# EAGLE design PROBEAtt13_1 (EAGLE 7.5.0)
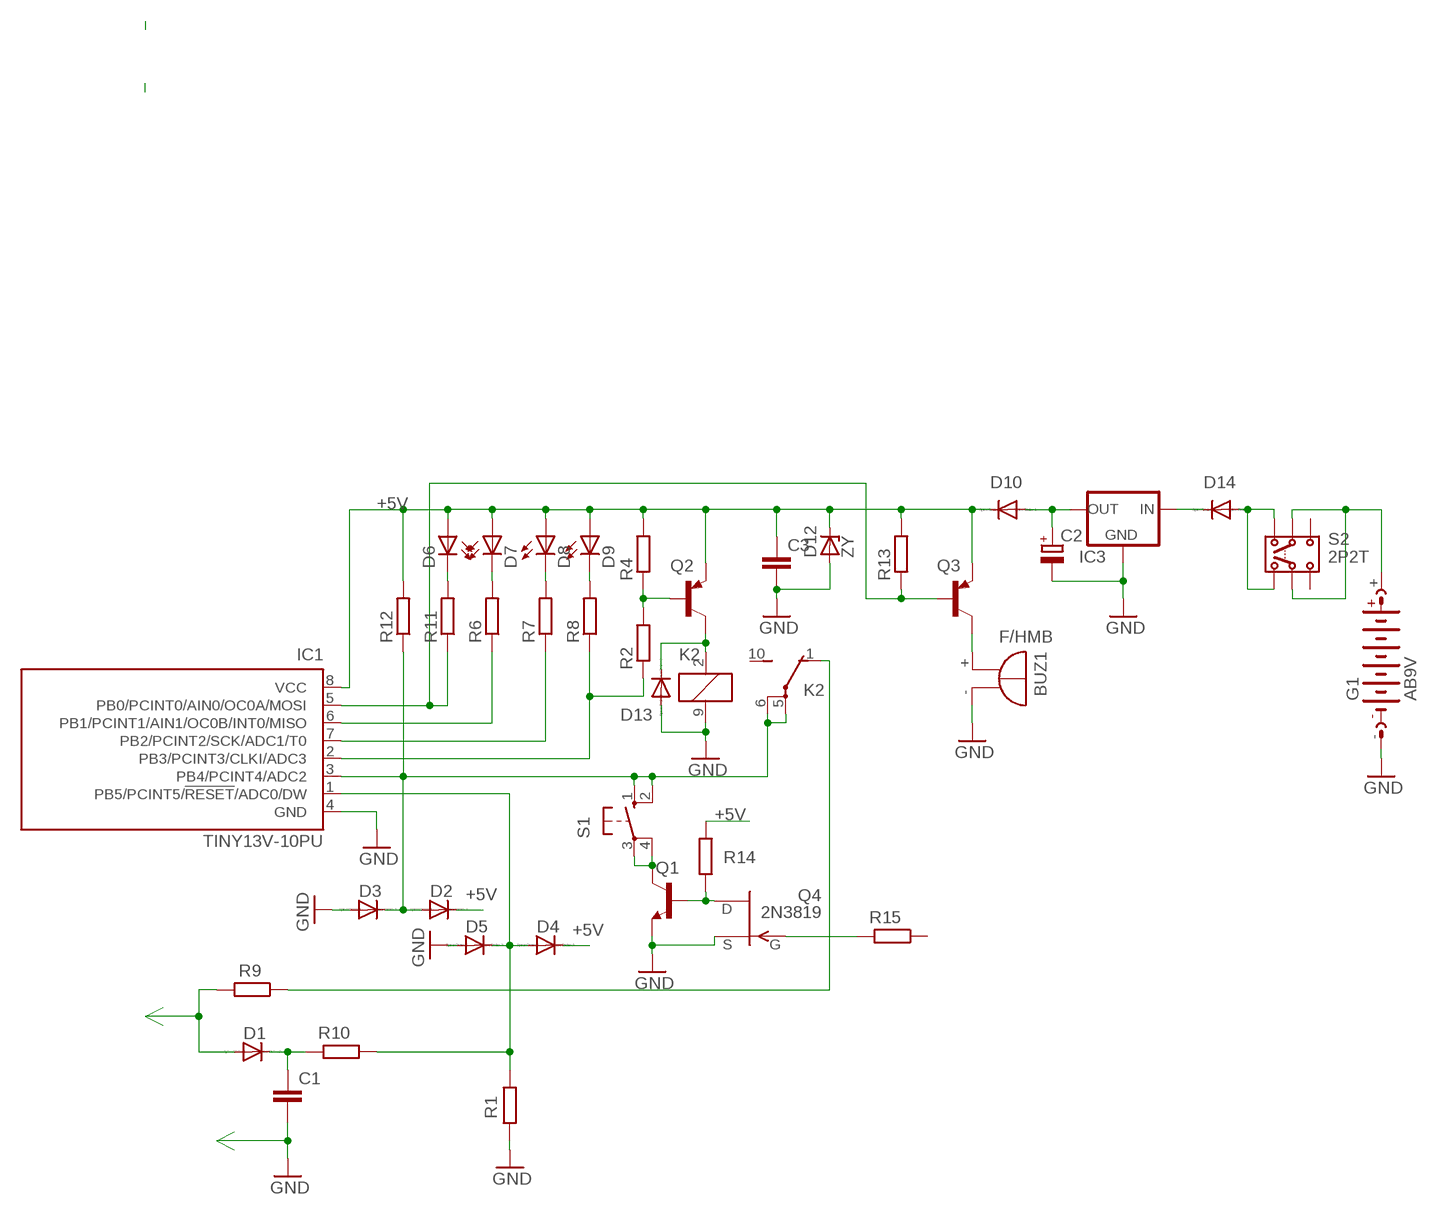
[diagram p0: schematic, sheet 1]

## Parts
BUZ1  F/HMB  [F/HMB]
C1  C-EU150-091X182  [C150-091X182]
C2  CPOL-EUE5-10.5  [E5-10,5]
C3  C-EUC1206  [C1206]
D1  1N4004  [DO41-10]
D2  1N4004  [DO41-10]
D3  1N4004  [DO41-10]
D4  1N4004  [DO41-10]
D5  1N4004  [DO41-10]
D6  LED5MM  [LED5MM]
D7  LED5MM  [LED5MM]
D8  LED5MM  [LED5MM]
D9  LED5MM  [LED5MM]
D10  1N4004  [DO41-10]
D12  ZY  [P1Z12]
D13  1N4004  [DO41-10]
D14  1N4004  [DO41-10]
G1  AB9V  [AB9V]
IC1  TINY13V-10PU  [DIL08]
IC3  78XXL  [78XXL]
K2  G5V1  [G5V1]
Q1  BC337  [TO92]
Q2  BC327  [TO92]
Q3  BC327  [TO92]
Q4  2N3819  [TO92]
R1  R-EU_0207/10  [0207/10]
R2  R-EU_0207/10  [0207/10]
R4  R-EU_0204/7  [0204/7]
R6  R-EU_0204/7  [0204/7]
R7  R-EU_0204/7  [0204/7]
R8  R-EU_0207/12  [0207/12]
R9  R-EU_0617/22  [0617/22]
R10  R-EU_0617/22  [0617/22]
R11  R-EU_0204/7  [0204/7]
R12  R-EU_0204/7  [0204/7]
R13  R-EU_0204/7  [0204/7]
R14  R-EU_0204/7  [0204/7]
R15  R-EU_0204/7  [0204/7]
S1  10-XX  [B3F-10XX]
S2  2P2T  [2P2T]

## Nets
+5V: C3.1 D2.C D4.C D6.A D7.A D8.A D9.A D10.C D12.C IC1.8(VCC) Q2.1(E) Q3.1(E) R4.2 R12.2 R13.2 R14.1
GND: BUZ1.- C1.2 C2.- C3.2 D3.A D5.A D12.A D13.A G1.- IC1.4(GND) IC3.GND K2.9 Q1.1(E) Q4.3(S) R1.2
N$1: IC1.5(PB0/PCINT0/AIN0/OC0A/MOSI) Q3.2(B) R11.1 R13.1
N$2: D6.K(C) R11.2
N$3: D2.A D3.C IC1.3(PB4/PCINT4/ADC2) K2.5(2:P) K2.6(2:P) R12.1 S1.1(S) S1.2(S1)
N$4: Q1.3(C) S1.3(P) S1.4(P1)
N$5: IC1.6(PB1/PCINT1/AIN1/OC0B/INT0/MISO) R6.1
N$6: D7.K(C) R6.2
N$7: IC1.7(PB2/PCINT2/SCK/ADC1/T0) R7.1
N$8: D8.K(C) R7.2
N$9: D4.A D5.C IC1.1(PB5/PCINT5/!RESET!/ADC0/DW) R1.1 R10.1
N$10: IC1.2(PB3/PCINT3/CLKI/ADC3) R2.1 R8.1
N$11: D9.K(C) R8.2
N$12: D13.C K2.2 Q2.3(C)
N$13: Q1.2(B) Q4.1(D) R14.2
N$14: C2.+ D10.A IC3.OUT
N$15: Q2.2(B) R2.2 R4.1
N$16: K2.1(2:O) R9.1
N$17: D1.A R9.2
N$18: D14.C IC3.IN
N$19: C1.1 D1.C R10.2
N$20: D14.A S2.1.1 S2.1.2
N$21: Q4.2(G) R15.2
N$22: G1.+ S2.2.1 S2.2.2
N$23: BUZ1.+ Q3.3(C)
Unconnected: K2.10(2:S) R15.1 S2.3.1 S2.3.2

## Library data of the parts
BUZ1 = buzzer:F/HMB: BUZZER; OC_FARNELL: unknown; OC_NEWARK: unknown
C1 C3 = rcl:C-EU: CAPACITOR, European symbol
C2 = rcl:CPOL-EU: POLARIZED CAPACITOR, European symbol
D1-D5 D10 D13 D14 = diode:1N4004: DIODE
D6-D9 = led:LED: LED
D12 = diode:ZY: Z DIODE
G1 = battery:AB9V: 9-V BATTERY CLIP
IC1 = atmel:TINY13: 8-bit AVR Microcontroller with 1K Bytes In-System Programmable Flash Source: http://www.atmel.com/dyn/resources/prod_documents/2535S.pdf; MPN: ATTINY13V-10PU; OC_FARNELL: 9171576; OC_NEWARK: 96K6523
IC3 = v-reg:78XXL: VOLTAGE REGULATOR
K2 = relay:G5V1: RELAY 1 x switch, 0.5 A/125 V AC, 1 A/24 V DC , Omron; MPN: G5V-1-DC24; OC_FARNELL: 9949593; OC_NEWARK: 36M6377
Q1 = transistor:BC337: NPN TRANSISTOR
Q2 Q3 = transistor-pnp:BC327: PNP Transistor
Q4 = transistor-fet:2N3819: N-Channel Junction FET
R1 R2 R4 R6-R15 = rcl:R-EU_: RESISTOR, European symbol
S1 = switch-omron:10-XX: OMRON SWITCH; MPN: B3F-1000; OC_FARNELL: 176432; OC_NEWARK: 36M3542
S2 = switch:2P2T: SLIDE SWITCH 2P2T Part No. SS-22F05-G(A)4 Source: CANAL ELECTRONIC CO., LTD .. switsch.pdf

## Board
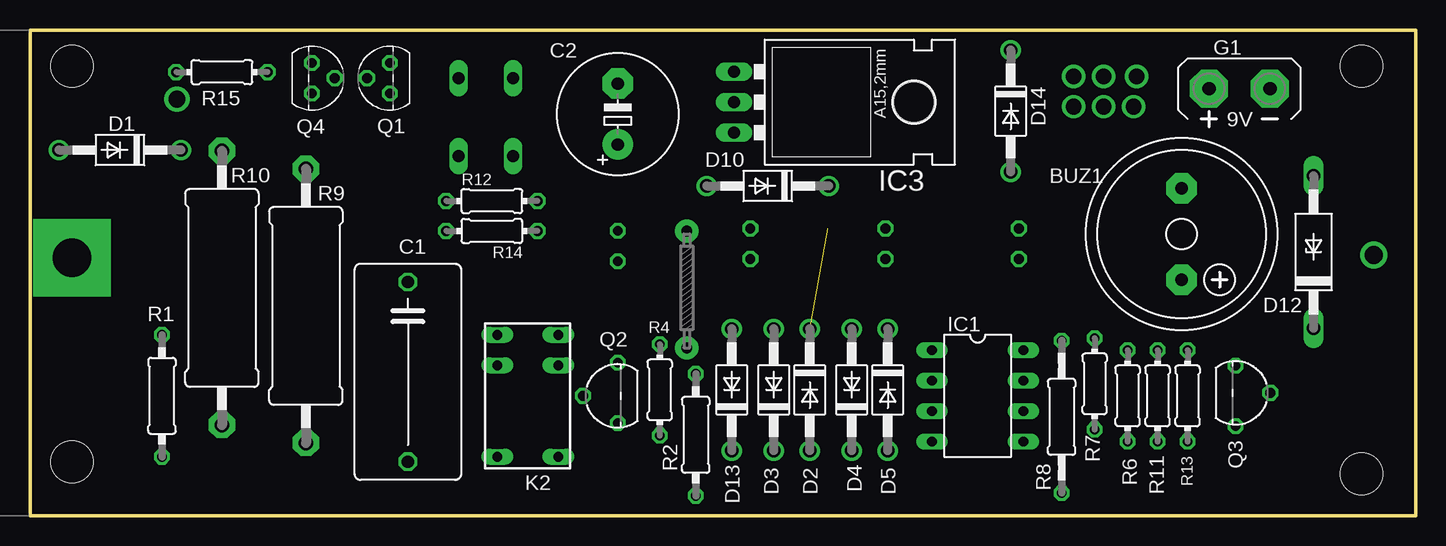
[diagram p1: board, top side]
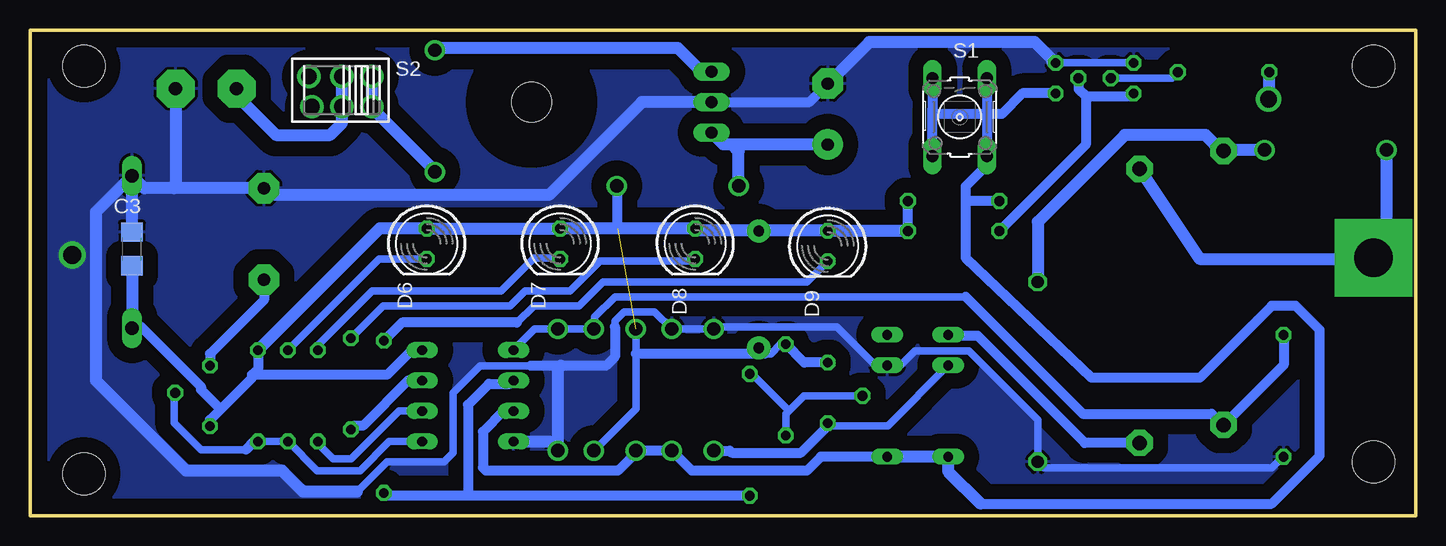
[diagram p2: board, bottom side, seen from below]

Size 115.5 x 40.5 mm. Coordinates in mm from the lower left corner, seen from the top.
Outline: 0,0 0,40.5 115.5,40.5 115.5,0 0,0
Copper layers (1*16): Top 0.035mm / dielectric 1.5mm / Bottom 0.035mm
Design rules "default": minimum track width 10mil, minimum drill 24mil, track to track 8mil, track to pad 8mil, pad to pad 8mil, via to via 8mil, smd to smd 8mil, copper to edge 40mil, drill to drill 8mil, minimum pad ring 10mil, minimum via ring 8mil, stop-mask expansion 4mil, vias tented up to drill 0mil, thermal gap 10mil
Holes 3.5 mm at 3.5,37.5 3.5,4.5 111,3.5 111,37.5

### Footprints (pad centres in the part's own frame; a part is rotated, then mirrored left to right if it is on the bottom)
F/HMB = drill 1.016 pad 2.54 octagon: + 3.81,0; - -3.81,0
C150-091X182 = drill 1.016 octagon: 1 -7.493,0; 2 7.493,0
E5-10,5 = drill 1.016 pad 2.54: + -2.54,0 | drill 1.016 pad 2.54 octagon: - 2.54,0
C1206 = smd 1.6 x 1.8: 1 -1.4,0; 2 1.4,0
DO41-10 = drill 1.118: A 5.08,0; C -5.08,0
LED5MM = drill 0.813 octagon: A -1.27,0; K 1.27,0
P1Z12 = drill 1.118 long: A 6.35,0; C -6.35,0
AB9V = drill 1.118 pad 3.15 octagon: + 0,2.54; - 0,-2.54
DIL08 = drill 0.813 long: 1 -3.81,-3.81; 2 -1.27,-3.81; 3 1.27,-3.81; 4 3.81,-3.81; 5 3.81,3.81; 6 1.27,3.81; 7 -1.27,3.81; 8 -3.81,3.81
78XXL = drill 1.016 long: GND 0,-3.81; IN -2.54,-3.81; OUT 2.54,-3.81 | hole 3.302: 0,11.176
G5V1 = drill 0.813 long: 1 -5.08,-2.54; 2 -2.54,-2.54; 5 5.08,-2.54; 6 5.08,2.54; 9 -2.54,2.54; 10 -5.08,2.54
TO92 = drill 0.813 octagon: 1 1.27,0; 2 0,1.905; 3 -1.27,0
TO92' = drill 0.813 octagon: 1 2.77,0; 2 0,2.905; 3 -2.27,0
0207/10 = drill 0.813 octagon: 1 -5.08,0; 2 5.08,0
0204/7 = drill 0.813 octagon: 1 -3.81,0; 2 3.81,0
0207/12 = drill 0.813 octagon: 1 -6.35,0; 2 6.35,0
0617/22 = drill 1.2 pad 2.184 octagon: 1 -11.43,0; 2 11.43,0
B3F-10XX = drill 1.016 long: 1 -3.251,2.261; 2 3.251,2.261; 3 -3.251,-2.261; 4 3.251,-2.261
2P2T = drill 1.3 pad 1.93: 1.1 -2.492,1.38; 1.2 -2.492,-1.126; 2.1 0,1.38; 2.2 0,-1.126; 3.1 2.492,1.38; 3.2 2.746,-1.126

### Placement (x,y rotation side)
BUZ1  96,23.5 270 top
C1  31.5,12 270 top
C2  49,33.5 90 top
C3  107,22.25 90 bottom
D1  7.5,30.5 180 top
D2  65,10.5 270 top
D3  62,10.5 90 top
D4  68.5,10.5 90 top
D5  71.5,10.5 270 top
D6  82.43,22.69 270 bottom
D7  71.31,22.69 270 bottom
D8  60.05,22.69 270 bottom
D9  49,22.5 270 bottom
D10  61.5,27.5 180 top
D12  107,22 90 top
D13  58.5,10.5 90 top
D14  81.75,33.75 270 top
G1  100.82,35.62 90 top
IC1  79,10 270 top
IC3  62.5,34.5 270 top
K2  41.5,10 270 top
Q1  30,36.5 90 top
Q2  BC327  [TO92']  49,10 90 top
Q3  BC327  [TO92']  100.5,10.25 270 top
Q4  23.5,36.5 270 top
R1  11,10 270 top
R2  55.5,6.75 90 top
R4  52.5,10.5 90 top
R6  91.5,10 90 top
R7  88.75,11 90 top
R8  86,8.25 90 top
R9  23,17.5 90 top
R10  16,19 90 top
R11  94,10 90 top
R12  38.5,26.25 0 top
R13  96.5,10 90 top
R14  38.5,23.75 180 top
R15  16,37 0 top
S1  38,33.25 270 bottom
S2  89.5,35.5 180 bottom

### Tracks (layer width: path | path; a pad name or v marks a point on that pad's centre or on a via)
+5V  (via drill 0.9 pad 1.93)  (1 unrouted)
  Bottom 0.61: D2.C 65,13.5 65,8.92 D4.C | R4.2 52.94,14.31 53.75,13.5 54.25,13.5
  Bottom 0.813: 59.86,23.77 D8.A | D10.C 66.58,24.04 66.5,23.96 | 65,13.5 54.25,13.5 v54.75,14 | 97,11.75 85.75,11.75 83.75,13.75 82.87,13.75 IC1.8 | R13.2 96.5,12.25 97,11.75 | Q2.1 50.96,12.77 R4.2 | D12.C 106.9,15.75 106.25,15.75 101.25,10.75 101.25,10.5 99.62,8.88 | v54.75,23.75 52.02,23.75 52,23.77 | R14.1 R12.2 | 48.98,23.75 D9.A | 97,11.75 97,11.5 99.62,8.88 | 99.62,8.88 100.5,8 Q3.1
  Bottom 1.016: D9.A 52,23.77 59.86,23.77 | D8.A 66.5,23.96 D7.A D6.A 86.35,23.96 R13.2 | C3.1 D12.C | R14.1 48.98,23.75
GND  (via drill 1.5)
  Bottom 0.61: Q4.3 Q1.1 30.27,37.77 | R1.2 11.08,4.92 12,4 30.99,4 C1.2 31.5,8 37.25,13.75 41.75,13.75 43,12.5 44,12.5 K2.9 45.04,12.54 48.25,15.75 58.33,15.75 D13.A D3.A 63.42,17 66,17 66.75,16.25 66.75,15.75 | IC1.4 72.27,6.19 D5.A | 73.75,12.5 78,12.5 80.25,10.25 80.25,5.25 81,4.5 85.75,4.5 88.25,2
  Bottom 0.813: 49.5,35.5 49.5,35.54 C2.- 50.54,34.5 IC3.GND | 66.75,15.75 66.75,13.25 67.5,12.5 71.25,12.5 73.75,12.5
  Bottom 1.016: IC1.4 72.19,6.19 71.5,5.5 71.5,12.25 71.25,12.5 | 88.25,2 92.75,2 94.5,3.75 102.5,3.75 110,11.25 110,25.35 107.42,27.93 | 107.42,27.93 D12.A 105.96,27.31 103.5,27.31 | 103.5,27.31 BUZ1.- 95.44,26.75 72.25,26.75 64.5,34.5 IC3.GND | G1.- 103.36,27.45 103.5,27.31 | C3.2 107,27.5 107.42,27.93 | 30.27,37.77 30.27,38.02 31.75,39.5 45.54,39.5 C2.-
  other vias: 112,21.75
  pour Bottom (isolate 1.27): 0.75,39.75 114.75,39.75 114.75,0.5 0.5,0.5 0.5,39.75
N$1
  Bottom 0.61: R13.1 R11.1 91.56,3.75 88,3.75 85.56,6.19 IC1.5 | 97.5,5.5 101.25,5.5 103.5,7.75 103.5,10.15 Q3.2
  Bottom 0.813: R13.1 96.81,6.19 97.5,5.5
N$2
  Bottom 0.61: D6.K 86.39,21.42 R11.2
N$3
  Bottom 0.813: IC1.3 76.02,8.73 77.75,7 77.75,4 77.5,3.75 66.5,3.75 65,5.25 D2.A D3.C 60.33,3.75 50.75,3.75 49.58,4.92 K2.6 | 37.5,26.5 37.5,21.5 27,11.5 18,11.5 12,17.5 10,17.5 8,15.5 8,5 12,1 36.25,1 | 37.5,26.5 37.5,27.49 35.74,29.25 S1.2 S1.1 | R12.1 37.25,26.25 37.5,26.5
  Bottom 1.016: K2.6 K2.5 38.96,3.71 36.25,1
N$4
  Bottom 0.813: Q1.3 32.77,35.23 34.5,33.5 40.25,33.5 40.25,34 | 40.25,34 S1.3 | S1.4 40.26,33.99 40.25,34
N$5
  Bottom 0.61: R6.1 91.5,6 90.25,4.75 88.75,4.75 84.75,8.75 82.83,8.75 IC1.6
N$6
  Bottom 0.61: D7.K 71.39,21.5 73.5,21.5 76.25,18.75 87,18.75 91.5,14.25 R6.2
N$7
  Bottom 0.813: IC1.7 83.98,11.27 87.75,7.5 88.44,7.5 R7.1
N$8
  Bottom 0.61: D8.K 60.22,21.25 68,21.25 70.5,18.75 74.25,18.75 75.5,17.5 86.06,17.5 R7.2
N$9
  Bottom 0.61: IC1.1 73.42,15.58 D5.C D4.A 68.42,15.58 68.42,16.58 66.75,18.25 37.5,18.25
  Bottom 0.813: R1.1 11,12.57 R10.1 15.93,7.5 16,7.5 17,8.5 27.75,8.5 37.5,18.25
N$10
  Bottom 0.813: IC1.2 75.46,11 77.25,11 79,9.25 79,1.92 78.75,1.67 | R2.1 78.75,1.67 | 78.75,1.67 85.77,1.67 R8.1
N$11
  Bottom 0.61: 74.9,16.1 73.5,17.5 69.75,17.5 67.75,19.5 50.73,19.5 D9.K
  Bottom 0.813: 74.9,16.1 84.5,16.1 R8.2
N$12
  Bottom 0.61: D13.C 58.42,5.42 | Q2.3 49,7.5 44,7.5 K2.2
  Bottom 0.813: 58.42,5.42 57.17,5.42 57,5.25 51.25,5.25 49,7.5
N$13
  Bottom 0.813: 27.5,35 23.73,35 Q4.1 | Q1.2 28.09,35.59 27.5,35 | 27.5,35 27.5,30.94 R14.2
N$14
  Bottom 1.016: C2.+ 57,30.96 | 57,30.96 57.69,30.96 IC3.OUT | D10.A 56.42,30.38 57,30.96
N$15
  Bottom 0.61: Q2.2 51,10 52.25,8.75 | 52.25,8.75 52.5,8.5 R4.1 | R2.2 55.33,11.83 52.25,8.75
N$16
  Bottom 0.813: R9.1 27.57,6.07 36.5,15 38.88,15 K2.1
N$17  (via drill 3.2 pad 6.45)
  Bottom 1.016: R9.2 17.99,21.42 4.58,21.42 4,22 v3.5,21.5 2.42,22.58 D1.A
N$18
  Bottom 1.016: IC3.IN 59.54,37.04 61.5,39 81.58,39 D14.C
N$19
  Bottom 1.016: C1.1 31.5,24.5 24.25,31.75 17.5,31.75 16.18,30.43 R10.2 15.93,30.5 D1.C
N$20
  Bottom 1.016: S2.1.2 S2.1.1 86.75,33.86 86.75,33.75 81.75,28.75 D14.A
N$21
  Bottom 0.61: Q4.2 20.31,36.5 R15.2
N$22
  Bottom 1.016: G1.+ 98.28,35.03 95,31.75 90.5,31.75 89.5,32.75 S2.2.1 S2.2.2
N$23
  Bottom 0.813: BUZ1.+ 96,18 100.5,13.5 Q3.3
N$24  (via drill 1.4)
  Bottom 1.016: 12.25,37 v12.25,34.75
